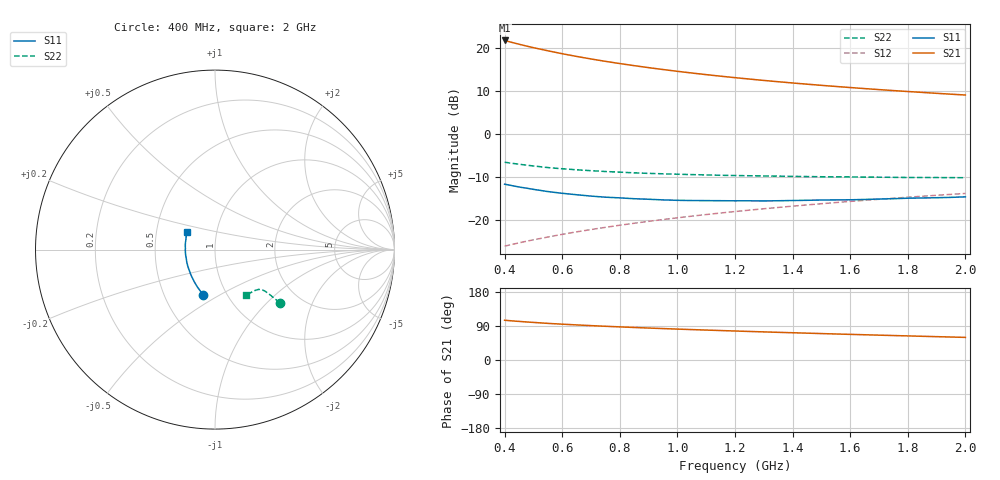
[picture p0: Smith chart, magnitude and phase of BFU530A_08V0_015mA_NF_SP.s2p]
! Filename:  P:\Prog\Test\Noise\ATS_data\Testdata_Net\06 Compressed Noise after Statistics\BFU530A_APG2013_33_A05_08p0V_015mA_NF_CM01_D.sf
! Date/Time: Tue 16/Apr/2013 15:10:58
! BFU530A_APG2013_33_A05_08p0V_1to25mA_NF_CM01_Bias6_R.sf
! Noise Parameter Data File
! BFU530A_APG2013_33_A05_08p0V_1to25mA_NF_CM01
! Date/time: Fri Apr 12 16:45:05 2013
! VAR V_out= 8.001000
! VAR I_out= 14.995000
! VAR V_in= 0.820500
! VAR I_in= 0.155000
! Device data file deembeded for feedlines and parallel
! Original file: \06 Compressed Noise after Statistics\BFU530A_APG2013_33_A05_08p0V_015mA_NF_CM01_R.sf
! Feed-files: PR017V01_150413_Feed1.s2p, PR017V01_150413_Feed2.s2p
! Parallel-file: PR017V01_150413_Par.s2p
# MHz S MA R 50
!  Freq-MHz  S11-mag  S11-arg  S21-mag  S21-arg  S12-mag  S12-arg  S22-mag  S22-arg
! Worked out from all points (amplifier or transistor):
!   37 points, 400 MHz to 2 GHz, reference 50 ohm
!   highest |S21| = 21.8 dB at 400 MHz (marker M1)
!   |S21| within 3 dB of that: start of sweep to 593.2 MHz
!   unconditionally stable (mu >= 1): 1.168 GHz to end of sweep
!   at 500 MHz: K = 0.88, MSG = 22.4 dB, |S12| = -24.7 dB
!   at 1.1 GHz: K = 1.00, MSG = 16.3 dB, |S12| = -18.8 dB
!   at 2 GHz: K = 1.00, MAG = 11.1 dB, |S12| = -13.9 dB
!   lowest NFmin = 0.90 dB at 420 MHz
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400  0.2586 -104.5  12.29 104.9  0.04893 68.8  0.4668 -39.2
420  0.2509 -107.2  11.78 103.6  0.05076 68.9  0.4559 -39.3
440  0.2434 -109.9  11.32 102.4  0.05258 69.1  0.4464 -39.4
460  0.2368 -112.3  10.89 101.3  0.05439 69.2  0.4378 -39.4
480  0.2313 -114.9  10.49 100.2  0.05622 69.4  0.4291 -39.4
500  0.2252 -117.2  10.12 99.2  0.05802 69.5  0.4218 -39.5
550  0.2122 -123.3  9.314 96.7  0.06251 69.9  0.404 -39.4
600  0.2024 -128.4  8.604 94.5  0.0672 70.2  0.3914 -39.4
650  0.1948 -133.4  8.001 92.6  0.07185 70.4  0.3808 -39.5
700  0.1879 -138.2  7.473 90.7  0.07647 70.6  0.3717 -39.6
750  0.1824 -142.7  7.01 89.0  0.08115 70.8  0.3635 -39.7
800  0.179 -147.1  6.606 87.4  0.08588 70.9  0.3573 -39.9
850  0.175 -151.5  6.244 85.8  0.09057 70.9  0.3508 -40.2
950  0.1696 -159.3  5.628 82.9  0.1001 70.9  0.3418 -40.8
1050  0.1667 -166.3  5.123 80.2  0.1096 70.8  0.3345 -41.5
1150  0.1659 -173.0  4.705 77.7  0.1192 70.5  0.3284 -42.5
1200  0.1655 -175.9  4.524 76.5  0.124 70.3  0.3265 -43.0
1350  0.1658 175.4  4.054 73.0  0.1385 69.7  0.321 -44.9
1500  0.169 167.5  3.679 69.7  0.153 69.0  0.3158 -46.9
1650  0.1716 160.9  3.372 66.6  0.1677 68.1  0.3131 -49.3
1750  0.1752 156.7  3.197 64.6  0.1773 67.4  0.3109 -50.8
2000  0.1841 147.5  2.836 59.7  0.2016 65.7  0.308 -55.3
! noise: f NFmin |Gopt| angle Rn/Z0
400  0.9664  0.1292  -168.7  0.0915
460  0.9356  0.1709  -172.8  0.0783
600  1.029  0.1431  -159.2  0.1016
800  0.9905  0.1706  -159.6  0.0883
1000  1.024  0.1898  -158.5  0.0831
1200  1.047  0.208  -150.6  0.0873
1400  1.074  0.2185  -146.7  0.0898
1600  1.088  0.2595  -141.3  0.0869
1800  1.076  0.277  -140.9  0.086
2000  1.101  0.2863  -138.2  0.0883
